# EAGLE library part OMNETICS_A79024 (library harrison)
Omnetics A79024 36-pin connector
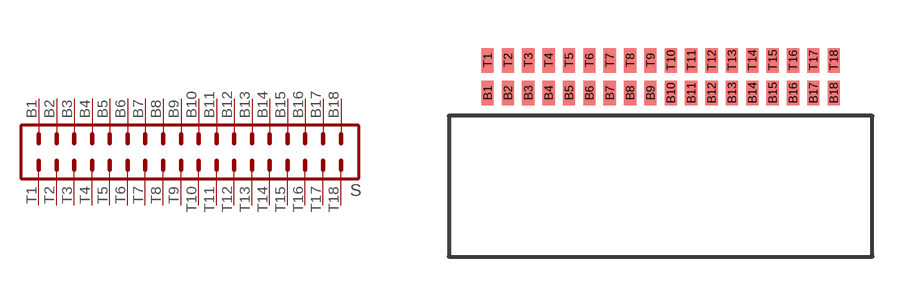
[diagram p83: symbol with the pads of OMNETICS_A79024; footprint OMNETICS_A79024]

Designator prefix S

## OMNETICS_A79024  [OMNETICS_A79024]
B1  B1  pas
B2  B2  pas
B3  B3  pas
B4  B4  pas
B5  B5  pas
B6  B6  pas
B7  B7  pas
B8  B8  pas
B9  B9  pas
B10  B10  pas
B11  B11  pas
B12  B12  pas
B13  B13  pas
B14  B14  pas
B15  B15  pas
B16  B16  pas
B17  B17  pas
B18  B18  pas
T1  T1  pas
T2  T2  pas
T3  T3  pas
T4  T4  pas
T5  T5  pas
T6  T6  pas
T7  T7  pas
T8  T8  pas
T9  T9  pas
T10  T10  pas
T11  T11  pas
T12  T12  pas
T13  T13  pas
T14  T14  pas
T15  T15  pas
T16  T16  pas
T17  T17  pas
T18  T18  pas

## Footprint OMNETICS_A79024 (pad centres in mm)
smd 0.381 x 0.762: B1 -5.397,0.711; B2 -4.763,0.711; B3 -4.128,0.711; B4 -3.493,0.711; B5 -2.857,0.711; B6 -2.223,0.711; B7 -1.587,0.711; B8 -0.953,0.711; B9 -0.318,0.711; B10 0.318,0.711; B11 0.953,0.711; B12 1.587,0.711; B13 2.223,0.711; B14 2.857,0.711; B15 3.493,0.711; B16 4.128,0.711; B17 4.763,0.711; B18 5.397,0.711; T1 -5.397,1.727; T2 -4.763,1.727; T3 -4.128,1.727; T4 -3.493,1.727; T5 -2.857,1.727; T6 -2.223,1.727; T7 -1.587,1.727; T8 -0.953,1.727; T9 -0.318,1.727; T10 0.318,1.727; T11 0.953,1.727; T12 1.587,1.727; T13 2.223,1.727; T14 2.857,1.727; T15 3.493,1.727; T16 4.128,1.727; T17 4.763,1.727; T18 5.397,1.727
